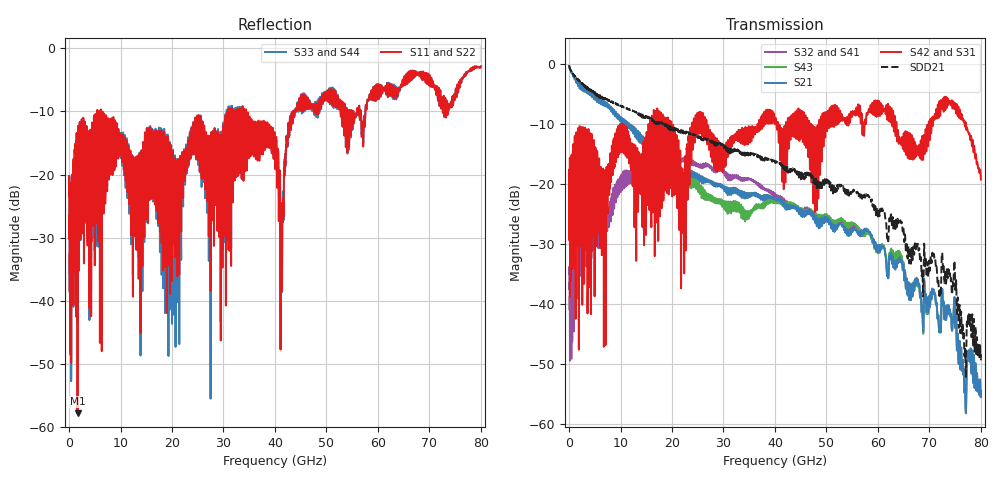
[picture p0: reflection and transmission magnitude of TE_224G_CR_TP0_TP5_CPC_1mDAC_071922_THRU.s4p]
!! Reference: tracy_3df_01a_2207
!! CHANNEL DESCRIPTION: TP0_TP5 CR Channel using 1meter DAC, CABLED CPC Host
!! MODEL DESCRIPTION: s4p, THRU
!! CONNECTOR DESCRIPTION: OSFP 200G OTB, CPC Socket
!! CABLE DESCRIPTION: 1meter 26AWG Cable
!! MODEL STATUS: Developmental
!! PORT DEFINITIONS:
!! Port  1  ----->  Side A  Side B  <-----  Port  2
!! Port  3  ----->  Side A  Side B  <-----  Port  4
# GHz S MA R 50
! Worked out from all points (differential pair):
!   8000 points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, 10 MHz to 80 GHz, reference 50 ohm
!   strongest paths, dB at 10 MHz, 20.01 GHz, 40.01 GHz, 60.01 GHz, 80 GHz:
!     S42: -24.6, -20.2, -10.1, -8.2, -19.3
!     S31: -24.6, -20.2, -10.1, -8.2, -19.3
!     S21: -0.4, -17.4, -22.6, -31.4, -55.1
!     S43: -0.4, -18.3, -23.1, -31.6, -55.0
!     S32: -34.9, -15.4, -21.8, -31.5, -55.1
!     S41: -34.9, -15.4, -21.8, -31.5, -55.1
!   taken as a pair (ports 1,3 in; 2,4 out), SDD21 dB: -0.3, -10.6, -16.3, -25.4, -49.0
!   lowest |S11| = -57.8 dB at 1.64 GHz (marker M1), VSWR 1.00, Z = 49.9 - j0.00388 ohm
!   |S11| at or under -10 dB: start of sweep to 5.488 GHz; 6.171 GHz to 30.97 GHz (24.8 GHz wide, 134 % of centre); 34.4 GHz to 43.55 GHz (9.158 GHz wide, 23.5 % of centre)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
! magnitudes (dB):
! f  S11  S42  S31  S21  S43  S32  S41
! 10 MHz  -23.3  -24.6  -24.6  -0.4  -0.4  -34.9  -34.9
! 1.64 GHz  -57.8  -19.6  -19.6  -2.7  -2.8  -33.3  -33.3
! 35.37 GHz  -12.0  -12.2  -12.2  -21.5  -24.4  -19.2  -19.2
! 41.35 GHz  -38.4  -16.6  -16.6  -23.2  -23.4  -22.2  -22.2
! 45.04 GHz  -7.4  -12.3  -12.3  -25.2  -25.1  -25.2  -25.2
! 73.57 GHz  -10.1  -5.8  -5.8  -41.4  -41.4  -41.4  -41.4
! 80 GHz  -2.9  -19.3  -19.3  -55.1  -55.0  -55.1  -55.1
